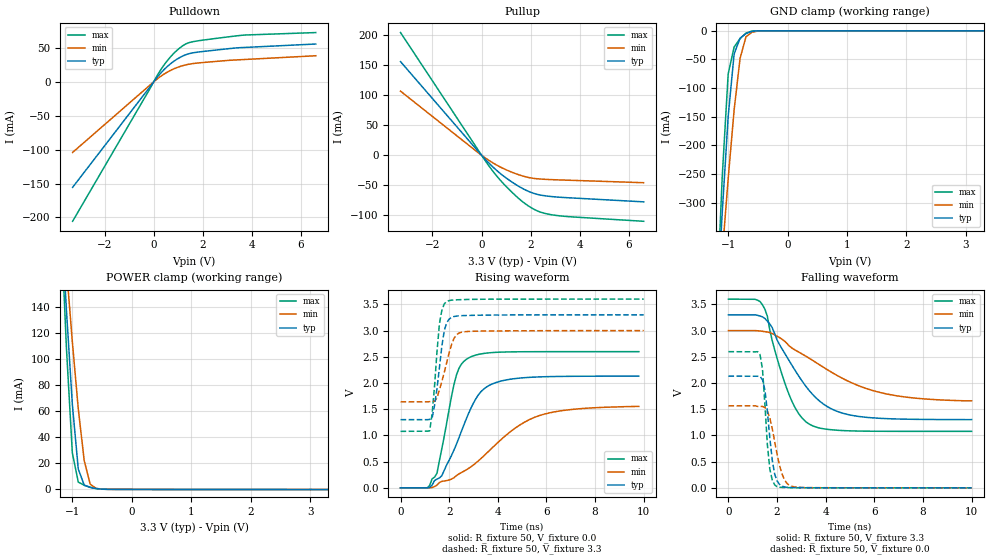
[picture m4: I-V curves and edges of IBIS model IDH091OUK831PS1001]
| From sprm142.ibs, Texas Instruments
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[Model]   IDH091OUK831PS1001
| I/O with pullup
Model_type   I/O
Vinh = 2.00
Vinl = 0.80
Enable   Active-Low
Polarity   Non-Inverting
| signals   A, GZ, Y
Vmeas = 1.5
|   typ   min   max
C_comp   1.4592p   1.4336p   1.5063p
|   typ   min   max
[Temperature Range]   25   -40   125
|   typ   min   max
[Voltage Range]   3.30V   3.00V   3.60V
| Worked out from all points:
|   slope of the pulldown table from 0 to 0.495 V, typ, clamps not added: 24 ohm
|   slope of the pullup table from 0 to 0.495 V, typ, clamps not added: 23.8 ohm
|   GND clamp passes 1 mA (typ) near -0.60 V on its own axis
|   POWER clamp passes 1 mA (typ) near -0.64 V on its own axis
|   rising waveform, R_fixture 50, V_fixture 0.0: 20-80 % time 1.22ns typ, 2.49ns min, 659ps max; typ from 0 V to 2.13 V
|   falling waveform, R_fixture 50, V_fixture 3.3: 20-80 % time 1.7ns typ, 3.02ns min, 1.01ns max; typ from 3.3 V to 1.3 V
|   rising waveform, R_fixture 50, V_fixture 3.3: 20-80 % time 327ps typ, 469ps min, 262ps max; typ from 1.3 V to 3.3 V
|   falling waveform, R_fixture 50, V_fixture 0.0: 20-80 % time 300ps typ, 432ps min, 239ps max; typ from 2.13 V to 0 V
[Pulldown]
|   Voltage   I(typ)   I(min)   I(max)
-3.3V     -155.6mA   -104.1mA   -205.6mA
200mV     9.243mA    5.866mA    12.7mA
600mV     24.13mA    15.28mA    33.3mA
800mV     29.87mA    18.87mA    41.37mA
1.1V      36.63mA    23.02mA    51.08mA
1.3V      39.97mA    25.04mA    55.82mA
1.6V      42.83mA    27mA       59.29mA
3.5V      50.44mA    32.65mA    68.4mA
6.6V      55.87mA    38.54mA    72.75mA
[GND_clamp]
|   Voltage   I(typ)   I(min)   I(max)
-3.3V     -4.927A    -3.712A    -6.4A
-1.2V     -505.6mA   -530mA     -497.3mA
-1.1V     -317.6mA   -390.7mA   -254.8mA
-1V       -149.8mA   -258.1mA   -75.21mA
-900mV    -40.36mA   -138.4mA   -28.31mA
-800mV    -13.04mA   -48.1mA    -13.49mA
-700mV    -4.677mA   -10.3mA    -3.929mA
-600mV    -901.8uA   -2.405mA   -447.5uA
-400mV    -4.618uA   -51.18uA   -472.4nA
3.3V      222pA      1.962uA    177.6pA
[Pullup]
|   Voltage   I(typ)   I(min)   I(max)
-3.3V     155.5mA    106.5mA    203.9mA
-200mV    9.306mA    6.233mA    12.42mA
300mV     -13.07mA   -8.546mA   -17.75mA
600mV     -24.68mA   -16mA      -33.65mA
900mV     -34.78mA   -22.33mA   -47.64mA
1.4V      -48.81mA   -30.78mA   -67.77mA
1.7V      -55.9mA    -34.78mA   -78.19mA
2V        -61.53mA   -37.68mA   -86.71mA
2.3V      -65.31mA   -39.22mA   -93.01mA
2.9V      -68.83mA   -40.61mA   -99.22mA
3.7V      -71.03mA   -41.73mA   -102.5mA
6.6V      -77.46mA   -45.65mA   -109.8mA
[POWER_clamp]
|   Voltage   I(typ)   I(min)   I(max)
-3.3V     2.116A     1.598A     2.746A
-1.2V     218.8mA    230.1mA    213.9mA
-1.1V     137.8mA    170.2mA    109mA
-1V       65.27mA    113.2mA    27.97mA
-900mV    15.59mA    61.69mA    5.615mA
-800mV    3.242mA    22.02mA    3.158mA
-700mV    1.508mA    4.028mA    1.661mA
-600mV    650uA      794.5uA    624uA
-500mV    185.1uA    185.9uA    140.5uA
3.3V      -108.3uA   -68.17uA   -162.1uA
[Ramp]
|   I(typ)   I(min)   I(max)
dV/dt_r   1.278/1.218n   0.933/2.485n   1.559/0.655n
dV/dt_f   1.199/1.705n   0.806/3.029n   1.513/1.012n
[Rising Waveform]
R_fixture = 50
V_fixture = 0.0
|  pu_on
|  TIME   V(typ)   V(min)   V(max)
0s        7nV        22nV       6nV
1.1ns     -96.84uV   -119.8uV   2.065mV
1.5ns     166.9mV    52.82mV    279.8mV
1.7ns     233.1mV    123.6mV    750.2mV
2.3ns     834.9mV    232.1mV    2.152V
2.8ns     1.421V     371.6mV    2.478V
3.2ns     1.774V     514.8mV    2.545V
3.6ns     1.942V     687.1mV    2.574V
5.6ns     2.114V     1.36V      2.597V
9.8ns     2.131V     1.554V     2.598V
[Falling Waveform]
R_fixture = 50
V_fixture = 3.3
V_fixture_min = 3.0
V_fixture_max = 3.6
|  pd_on
|  TIME   V(typ)   V(min)   V(max)
0s        3.3V       3V         3.6V
1.4ns     3.262V     2.987V     3.49V
1.8ns     3.057V     2.943V     2.81V
2.5ns     2.424V     2.707V     1.772V
2.9ns     2.125V     2.588V     1.408V
3.4ns     1.815V     2.45V      1.197V
4.2ns     1.516V     2.217V     1.11V
5.2ns     1.373V     1.977V     1.085V
7.1ns     1.312V     1.744V     1.078V
10ns      1.302V     1.66V      1.078V
[Rising Waveform]
R_fixture = 50
V_fixture = 3.3
V_fixture_min = 3.0
V_fixture_max = 3.6
|  pd_off
|  TIME   V(typ)   V(min)   V(max)
0s        1.301V     1.64V      1.078V
1.2ns     1.306V     1.644V     1.087V
1.3ns     1.332V     1.649V     1.417V
1.4ns     1.576V     1.648V     1.947V
1.6ns     2.293V     1.869V     3.13V
1.8ns     3.002V     2.205V     3.51V
1.9ns     3.15V      2.393V     3.556V
2.2ns     3.268V     2.851V     3.584V
2.6ns     3.286V     2.976V     3.592V
10ns      3.3V       3V         3.6V
[Falling Waveform]
R_fixture = 50
V_fixture = 0.0
|  pu_off
|  TIME   V(typ)   V(min)   V(max)
0s        2.131V     1.565V     2.598V
1.3ns     2.126V     1.555V     2.541V
1.4ns     2.061V     1.552V     2.264V
1.5ns     1.868V     1.532V     1.59V
1.7ns     960.6mV    1.335V     362.8mV
1.8ns     535.5mV    1.133V     153mV
2ns       131.8mV    640.6mV    23.27mV
2.3ns     18.18mV    157.8mV    6.556mV
2.7ns     5.596mV    19.75mV    3.109mV
10ns      2.534uV    61.76uV    1.481uV
